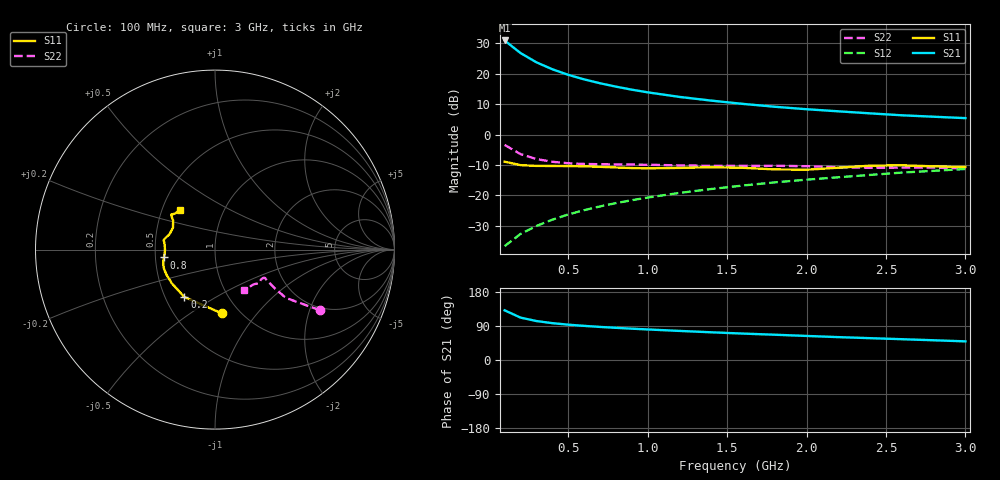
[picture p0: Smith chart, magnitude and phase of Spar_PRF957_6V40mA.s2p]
! Filename:  PRF957R.S2P  Version:  3.0
! NXP part #:  PRF957  Date:  Nov 1998
! Bias condition:  Vce=6V, Ic=40mA
#  MHz  S  MA  R 50
! Freq  S11  S21  S12  S22
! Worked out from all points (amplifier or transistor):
!   20 points, 100 MHz to 3 GHz, reference 50 ohm
!   highest |S21| = 31.0 dB at 100 MHz (marker M1)
!   |S21| within 3 dB of that: start of sweep to 172.4 MHz
!   unconditionally stable (mu >= 1): 541.3 MHz to end of sweep
!   at 400 MHz: K = 0.97, MSG = 24.7 dB, |S12| = -28.0 dB
!   at 1.2 GHz: K = 1.05, MAG = 14.4 dB, |S12| = -19.2 dB
!   at 3 GHz: K = 1.03, MAG = 7.4 dB, |S12| = -11.3 dB
!   lowest NFmin = 2.10 dB at 500 MHz
!   S11 on the Smith chart (normalised r, x): 100 MHz: 0.83, -0.68; 200 MHz: 0.63, -0.37; 800 MHz: 0.56, -0.05; 3 GHz: 0.62, +0.30
100  0.3582 -83.6  35.28 131.1  0.01461 69.2  0.676 -30.0
200  0.3145 -122.9  21.9 111.9  0.0232 69.6  0.4779 -34.3
300  0.3052 -142.0  15.44 102.8  0.03138 72.1  0.3953 -32.9
400  0.3043 -152.6  11.86 97.2  0.03984 74.3  0.3569 -31.4
500  0.3038 -159.2  9.615 93.2  0.04851 75.8  0.3378 -30.6
600  0.3006 -163.7  8.091 90.1  0.05709 76.8  0.3286 -30.2
700  0.295 -167.5  6.984 87.4  0.06581 77.4  0.325 -30.0
800  0.2879 -171.3  6.144 84.9  0.07452 77.8  0.3234 -29.8
900  0.2815 -175.3  5.476 82.7  0.08325 78.1  0.3214 -29.6
1000  0.2785 -179.5  4.95 80.6  0.09205 78.2  0.3188 -29.6
1200  0.2831 173.5  4.162 76.8  0.1098 78.0  0.3111 -30.5
1400  0.2906 169.6  3.618 73.1  0.1272 77.6  0.3058 -33.1
1600  0.2839 166.8  3.194 69.7  0.1452 77.1  0.3067 -35.8
1800  0.2675 161.4  2.867 66.7  0.1636 76.3  0.3073 -37.5
2000  0.2643 152.3  2.611 63.5  0.1812 75.8  0.3015 -38.8
2200  0.2851 145.0  2.412 60.4  0.1986 75.0  0.2906 -41.6
2400  0.3079 142.3  2.232 57.6  0.2169 74.0  0.2844 -45.7
2600  0.3126 141.3  2.075 54.9  0.237 72.9  0.2857 -49.5
2800  0.3 138.2  1.965 52.0  0.2535 72.3  0.2856 -51.8
3000  0.2936 130.9  1.864 49.2  0.2715 71.6  0.2779 -53.9
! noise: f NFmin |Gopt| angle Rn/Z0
500  2.1  0.29  -129  0.13
800  2.4  0.28  178  0.1
900  2.46  0.36  173  0.08
1000  2.6  0.2  155  0.22
1500  2.89  0.39  -133  0.28
2000  2.89  0.39  -133  0.28
